[IBIS Ver]   3.2
[File Name]   sprm191a.ibs
[File Rev]   0.1
[Date]   April 20, 2006
[Source]   File Originated at Texas Instruments
[Disclaimer]   Please be aware that in the absence of a written agreement
|   Texas Instruments(TI) assumes no liability for:
|   (1) The accuracy of the IBIS models provided to your company
|   (2) The proper functioning of these Models in your design
|   or for any resulting applications;or
|   (3) Infringement of patents,copyrights, or intellectual
|   property rights resulting from your use of these models.
|   TI provides IBIS Models as a service to our customers and
|   therefore reserves the right to limit distribution of the
|   Models.
[Copyright]   Property of Texas Instruments Incorporated.
|   Unauthorized reproduction and/or distribution is strictly
|   prohibited.
|   This product is protected under copyright law and trade
|   secret law as an unpublished work.
|   Created 1999,(C) Copyright 1999-2000,
|   Texas Instruments Incorporated., All Rights Reserved.
|   These commodities are under the U.S.
|   Government distribution license control.As such,they are not
|   to be re-exported without the prior approval of the U.S.
|   Department of Commerce.
[Component]   c6727_gdh
[Manufacturer]   Texas Instruments
[Package]
|Variable   Typ   Min   Max
R_pkg   3.500e-01   2.78346e-01  4.67972e-01
L_pkg   4.000e-09   2.63574e-09  6.33212e-09
C_pkg   4.300e-013  3.00224E-013 6.87584E-013
[Pin]   signal_name   model_name
C2   AHCLKX0   BC3325BSHY
C1   AMUTE0   BC3325BSHY
C3   HD[23]   BC3325BSHYPD
D2   AMUTE1   BC3325BSHY
D1   AHCLKX1   BC3325BSHY
D3   HD[22]   BC3325BSHYPD
E2   ACLKX1   BC3325BSHY
E1   ACLKR1   BC3325BSHY
E3   HD[21]   BC3325BSHYPD
F2   AFSX1   BC3325BSHY
F1   AFSR1   BC3325BSHY
F4   HD[20]   BC3325BSHYPD
F3   HD[19]   BC3325BSHYPD
G2   RESET   IC33SHY
G4   HD[18]   BC3325BSHYPD
G3   HD[17]   BC3325BSHYPD
H2   CLKIN   IC33SHY
H1   HD[16]   BC3325BSHYPD
H4   HD[31]   BC3325BSHYPD
K3   TMS   IC33SHYPU
K4   TRST   IC33SPD
L2   HD[30]   BC3325BSHYPD
L1   TDI   IC33SHYPU
M2   TDO   BC3325BSHYPU
L4   HD[29]   BC3325BSHYPD
L3   HD[28]   BC3325BSHYPD
M1   EMU0   BC3325BSHYPU
M3   HD[27]   BC3325BSHYPD
N3   HD[26]   BC3325BSHYPD
N1   EMU1   BC3325BSHYPU
N2   HD[25]   BC3325BSHYPD
P1   TCK   IC33SHYPU
P2   HD[24]   BC3325BSHYPD
R2   EM_D[23]   BC3325BSHYPD
N4   EM_D[22]   BC3325BSHYPD
R3   SDRAM_CAS   BC3325BSHY
P3   EM_D[21]   BC3325BSHYPD
T3   EM_WE   BC3325BSHY
R4   EM_WE_DQM[0]   BC3325BSHY
P4   EM_D[20]   BC3325BSHYPD
T4   EM_D[7]   BC3325BSHY
R5   EM_D[6]   BC3325BSHY
P5   EM_D[19]   BC3325BSHYPD
T5   EM_D[5]   BC3325BSHY
R6   EM_D[4]   BC3325BSHY
N6   EM_D[18]   BC3325BSHYPD
P6   EM_D[17]   BC3325BSHYPD
T6   EM_D[3]   BC3325BSHY
R7   EM_D[2]   BC3325BSHY
N7   EM_D[16]   BC3325BSHYPD
P7   EM_D[31]   BC3325BSHYPD
R8   EM_D[1]   BC3325BSHY
T8   EM_D[0]   BC3325BSHY
N8   EM_D[30]   BC3325BSHYPD
N9   EM_D[29]   BC3325BSHYPD
R9   EM_D[15]   BC3325BSHY
T9   EM_D[14]   BC3325BSHY
P9   EM_D[28]   BC3325BSHYPD
N10   EM_D[27]   BC3325BSHYPD
R10   EM_D[13]   BC3325BSHY
R11   EM_D[12]   BC3325BSHY
T11   EM_D[11]   BC3325BSHY
R12   EM_D[10]   BC3325BSHY
T12   EM_D[9]   BC3325BSHY
R13   EM_D[8]   BC3325BSHY
T13   EM_WE_DQM[1]   BC3325BSHY
R14   EM_CLK   BC3325BSHY
T14   EM_SDCKE   BC3325BSHY
P12   EM_A[12]   BC3325BSHYPD
P10   EM_D[26]   BC3325BSHYPD
N11   EM_D[25]   BC3325BSHYPD
P11   EM_D[24]   BC3325BSHYPD
P13   EM_WE_DQM[2]   BC3325BSHYPU
R15   EM_WE_DQM[3]   BC3325BSHYPU
P14   HD[7]   BC3325BSHYPD
P15   EM_A[11]   BC3325BSHY
N14   HD[6]   BC3325BSHYPD
P16   EM_A[9]   BC3325BSHY
N15   EM_A[8]   BC3325BSHY
N13   HD[5]   BC3325BSHYPD
N16   EM_A[7]   BC3325BSHY
M15   EM_A[6]   BC3325BSHY
L14   HD[4]   BC3325BSHYPD
M16   EM_A[5]   BC3325BSHY
L15   EM_A[4]   BC3325BSHY
L13   HD[3]   BC3325BSHYPD
M14   HD[2]   BC3325BSHYPD
L16   EM_A[3]   BC3325BSHY
K15   EM_A[2]   BC3325BSHY
K14   HD[1]   BC3325BSHYPD
K13   HD[0]   BC3325BSHYPD
J15   EM_A[1]   BC3325BSHY
J16   EM_A[0]   BC3325BSHY
J13   HD[15]   BC3325BSHYPD
H13   HD[14]   BC3325BSHYPD
H15   EM_A[10]   BC3325BSHY
H16   EM_BA[1]   BC3325BSHY
H14   HD[13]   BC3325BSHYPD
G13   HD[12]   BC3325BSHYPD
G15   EM_BA[0]   BC3325BSHY
F15   EM_CS[0]   BC3325BSHY
G14   HD[11]   BC3325BSHYPD
F16   SDRAM_RAS   BC3325BSHY
E15   EM_CS[1]   BC3325BSHY
F13   HD[10]   BC3325BSHYPD
E16   EM_RNW   BC3325BSHY
D15   EM_OE   BC3325BSHY
F14   HD[9]   BC3325BSHYPD
D16   SPI0_ENA   BC3325BSHY
E14   HD[8]   BC3325BSHYPD
C15   SPI0_SCS   BC3325BSHY
D14   EM_WAIT   BC3325BSHYPU
C16   SPI0_SCLK   BC3325BSHY
C14   AHCLKR2   BC3325BSHYPD
C13   ACLKR2   BC3325BSHYPD
C12   AFSR2   BC3325BSHYPD
B15   SPI0_SIMO   BC3325BSHY
B14   SPI0_SOMI   BC3325BSHY
A14   AXR0[0]   BC3325BSHY
B13   AXR0[1]   BC3325BSHY
A13   AXR0[2]   BC3325BSHY
B12   AXR0[3]   BC3325BSHY
D11   ACLKX2   BC3325BSHYPD
A12   AXR0[4]   BC3325BSHY
B11   AXR0[5]   BC3325BSHY
C11   AFSX2   BC3325BSHYPD
D10   AMUTE2   BC3325BSHYPD
A11   AXR0[6]   BC3325BSHY
B10   AXR0[7]   BC3325BSHY
C10   HCNTL1   BC3325BSHYPD
D9   HCNTL0   BC3325BSHYPD
B9   AXR0[8]   BC3325BSHY
A9   AXR0[9]   BC3325BSHY
C9   HAS   BC3325BSHYPD
D8   HRWN   BC3325BSHYPD
B8   AXR0[10]   BC3325BSHY
A8   AXR0[11]   BC3325BSHY
C8   HCS   BC3325BSHYPU
D7   HDS1   BC3325BSHYPU
B7   AXR0[12]   BC3325BSHY
B6   AXR0[13]   BC3325BSHY
C7   HDS2   BC3325BSHYPU
A6   AXR0[14]   BC3325BSHY
B5   AXR0[15]   BC3325BSHY
D6   HRDY   BC3325BSHYPD
A5   ACLKR0   BC3325BSHY
B4   AFSR0   BC3325BSHY
C6   HBE[0]   BC3325BSHYPD
A4   ACLKX0   BC3325BSHY
C5   HBE[1]   BC3325BSHYPD
B3   AHCLKR0   BC3325BSHY
C4   HBE[2]   BC3325BSHYPD
A3   AFSX0   BC3325BSHY
B2   HBE[3]   BC3325BSHYPD
[Package Model]   BGA
[Define Package Model]  BGA
[Manufacturer]   Texas Instruments
[OEM]   Texas Instruments
[Description]   BGA
[Number Of Sections]  1
[Number Of Pins]  152
[Pin Numbers]
C2   Len=0  R=0.339392   L=3.99674e-09  C=4.70683E-013 /
C1   Len=0  R=0.387574   L=4.72766e-09  C=4.57896E-013 /
C3   Len=0  R=0.354062   L=4.32098e-09  C=4.78888E-013 /
D2   Len=0  R=0.355048   L=4.40226e-09  C=4.28982E-013 /
D1   Len=0  R=0.373336   L=5.0292e-09   C=4.24207E-013 /
D3   Len=0  R=0.33615   L=4.05326e-09  C=4.47644E-013 /
E2   Len=0  R=0.340312   L=3.9161e-09   C=4.31444E-013 /
E1   Len=0  R=0.37303   L=4.38348e-09  C=4.04001E-013 /
E3   Len=0  R=0.317216   L=3.59786e-09  C=4.63371E-013 /
F2   Len=0  R=0.349102   L=3.8723e-09   C=3.79014E-013 /
F1   Len=0  R=0.387412   L=4.62594e-09  C=3.44324E-013 /
F4   Len=0  R=0.302866   L=3.27248e-09  C=4.13775E-013 /
F3   Len=0  R=0.309298   L=3.60524e-09  C=4.51108E-013 /
G2   Len=0  R=0.40644   L=4.74502e-09  C=4.38027E-013 /
G4   Len=0  R=0.323936   L=3.67236e-09  C=5.59319E-013 /
G3   Len=0  R=0.363316   L=4.41228e-09  C=4.25543E-013 /
H2   Len=0  R=0.331636   L=4.17322e-09  C=3.77069E-013 /
H1   Len=0  R=0.3734   L=4.74898e-09  C=3.37117E-013 /
H4   Len=0  R=0.305394   L=3.38732e-09  C=4.11321E-013 /
K3   Len=0  R=0.34395   L=4.19168e-09  C=4.19243E-013 /
K4   Len=0  R=0.323068   L=3.56512e-09  C=4.53466E-013 /
L2   Len=0  R=0.415648   L=4.82438e-09  C=4.10039E-013 /
L1   Len=0  R=0.36658   L=4.26388e-09  C=3.37108E-013 /
M2   Len=0  R=0.351496   L=3.77214e-09  C=4.40172E-013 /
L4   Len=0  R=0.29318   L=3.0961e-09   C=4.23678E-013 /
L3   Len=0  R=0.303374   L=3.5041e-09   C=3.70824E-013 /
M1   Len=0  R=0.381336   L=4.89728e-09  C=3.42681E-013 /
M3   Len=0  R=0.30869   L=3.78928e-09  C=4.25211E-013 /
N3   Len=0  R=0.354404   L=4.79456e-09  C=4.88341E-013 /
N1   Len=0  R=0.377298   L=5.26052e-09  C=3.88177E-013 /
N2   Len=0  R=0.354446   L=4.67068e-09  C=4.40298E-013 /
P1   Len=0  R=0.39216   L=5.42366e-09  C=4.70847E-013 /
P2   Len=0  R=0.33903   L=4.33112e-09  C=4.85018E-013 /
R2   Len=0  R=0.358758   L=4.69614e-09  C=5.20436E-013 /
P3   Len=0  R=0.317008   L=3.1663e-09   C=5.79127E-013 /
R3   Len=0  R=0.377564   L=4.6553e-09   C=5.21684E-013 /
P4   Len=0  R=0.334572   L=4.1666e-09   C=5.00816E-013 /
T3   Len=0  R=0.39423   L=4.83226e-09  C=4.65868E-013 /
R4   Len=0  R=0.348864   L=4.1244e-09   C=4.5167E-013 /
P5   Len=0  R=0.318642   L=3.77818e-09  C=4.86875E-013 /
T4   Len=0  R=0.383618   L=4.47018e-09  C=4.83017E-013 /
R5   Len=0  R=0.340902   L=3.80248e-09  C=4.68627E-013 /
N6   Len=0  R=0.338592   L=4.07018e-09  C=5.02179E-013 /
T5   Len=0  R=0.377266   L=4.8863e-09   C=4.05001E-013 /
R6   Len=0  R=0.396836   L=4.96212e-09  C=4.46027E-013 /
P6   Len=0  R=0.284454   L=3.0839e-09   C=4.56304E-013 /
N7   Len=0  R=0.343606   L=4.04324e-09  C=5.01509E-013 /
T6   Len=0  R=0.367898   L=4.60384e-09  C=3.44563E-013 /
R7   Len=0  R=0.382064   L=4.85522e-09  C=4.38861E-013 /
P7   Len=0  R=0.304548   L=3.55168e-09  C=5.16335E-013 /
N8   Len=0  R=0.345366   L=4.34114e-09  C=4.66695E-013 /
R8   Len=0  R=0.374476   L=4.38938e-09  C=4.34623E-013 /
T8   Len=0  R=0.349502   L=4.05058e-09  C=3.23466E-013 /
N9   Len=0  R=0.286356   L=2.93566e-09  C=4.56363E-013 /
R9   Len=0  R=0.31836   L=3.642e-09   C=4.12715E-013 /
T9   Len=0  R=0.35189   L=4.19304e-09  C=3.70599E-013 /
P9   Len=0  R=0.286986   L=3.13788e-09  C=4.011E-013 /
N10  Len=0  R=0.298736   L=3.01978e-09  C=4.59479E-013 /
R10  Len=0  R=0.308532   L=3.57838e-09  C=4.08798E-013 /
R11  Len=0  R=0.307654   L=3.53184e-09  C=4.41997E-013 /
T11  Len=0  R=0.347386   L=4.44308e-09  C=4.11649E-013 /
R12  Len=0  R=0.326916   L=3.9885e-09   C=4.6626E-013 /
T12  Len=0  R=0.355142   L=4.45764e-09  C=4.33576E-013 /
R13  Len=0  R=0.336044   L=4.09862e-09  C=4.60055E-013 /
T13  Len=0  R=0.37393   L=4.23852e-09  C=4.58815E-013 /
R14  Len=0  R=0.351614   L=4.08646e-09  C=5.28565E-013 /
T14  Len=0  R=0.37809   L=4.5564e-09   C=4.93324E-013 /
P12  Len=0  R=0.297444   L=3.53228e-09  C=4.63846E-013 /
P10  Len=0  R=0.39935   L=5.59426e-09  C=6.87584E-013 /
N11  Len=0  R=0.355874   L=4.34494e-09  C=6.3559E-013 /
P11  Len=0  R=0.39247   L=5.28174e-09  C=6.34721E-013 /
P13  Len=0  R=0.398214   L=5.2647e-09   C=5.91166E-013 /
R15  Len=0  R=0.41964   L=4.4944e-09   C=5.41393E-013 /
P14  Len=0  R=0.353802   L=4.03244e-09  C=4.63753E-013 /
P15  Len=0  R=0.390764   L=4.98794e-09  C=5.13753E-013 /
N14  Len=0  R=0.383586   L=4.80594e-09  C=5.39901E-013 /
P16  Len=0  R=0.414816   L=5.00038e-09  C=4.07424E-013 /
N15  Len=0  R=0.435388   L=5.30096e-09  C=4.54764E-013 /
M14  Len=0  R=0.400542   L=5.23214e-09  C=5.86961E-013 /
N16  Len=0  R=0.405086   L=5.0574e-09   C=3.23989E-013 /
M15  Len=0  R=0.42635   L=5.33792e-09  C=4.20074E-013 /
L13  Len=0  R=0.309456   L=3.72312e-09  C=4.32031E-013 /
M16  Len=0  R=0.400858   L=5.16958e-09  C=3.79026E-013 /
L15  Len=0  R=0.356984   L=4.67638e-09  C=4.12267E-013 /
L14  Len=0  R=0.390396   L=5.13432e-09  C=5.45077E-013 /
K13  Len=0  R=0.440966   L=6.33212e-09  C=5.175E-013 /
L16  Len=0  R=0.3967   L=5.2994e-09   C=3.29066E-013 /
K15  Len=0  R=0.400428   L=4.8064e-09   C=4.2299E-013 /
K14  Len=0  R=0.43253   L=5.39866e-09  C=5.07689E-013 /
J13  Len=0  R=0.397262   L=4.91252e-09  C=4.7853E-013 /
J15  Len=0  R=0.334622   L=3.60426e-09  C=3.60659E-013 /
J16  Len=0  R=0.366318   L=4.17084e-09  C=3.68789E-013 /
H13  Len=0  R=0.296514   L=2.63574e-09  C=3.47293E-013 /
H15  Len=0  R=0.347474   L=3.63696e-09  C=3.6496E-013 /
H16  Len=0  R=0.387966   L=4.62782e-09  C=3.56703E-013 /
H14  Len=0  R=0.314584   L=3.5549e-09   C=4.15173E-013 /
G13  Len=0  R=0.292528   L=3.00696e-09  C=3.79816E-013 /
G15  Len=0  R=0.336178   L=3.8189e-09   C=4.0186E-013 /
F15  Len=0  R=0.373872   L=4.34952e-09  C=4.80159E-013 /
G14  Len=0  R=0.322406   L=3.52692e-09  C=4.7568E-013 /
F16  Len=0  R=0.398476   L=4.75114e-09  C=4.24914E-013 /
E15  Len=0  R=0.370362   L=4.30076e-09  C=4.56163E-013 /
F13  Len=0  R=0.307978   L=3.2259e-09   C=4.49248E-013 /
E16  Len=0  R=0.431744   L=4.6978e-09   C=4.0359E-013 /
D15  Len=0  R=0.441372   L=4.83302e-09  C=4.80547E-013 /
F14  Len=0  R=0.322668   L=3.63798e-09  C=4.62158E-013 /
D16  Len=0  R=0.400788   L=4.68854e-09  C=4.4558E-013 /
E14  Len=0  R=0.322534   L=3.70792e-09  C=4.33147E-013 /
C15  Len=0  R=0.371338   L=4.73808e-09  C=4.46122E-013 /
D14  Len=0  R=0.340548   L=3.98704e-09  C=4.30597E-013 /
C16  Len=0  R=0.418262   L=5.5125e-09   C=4.62327E-013 /
C14  Len=0  R=0.358998   L=4.33078e-09  C=4.82489E-013 /
C13  Len=0  R=0.32407   L=3.70724e-09  C=5.51319E-013 /
C12  Len=0  R=0.304854   L=3.50414e-09  C=5.56124E-013 /
B15  Len=0  R=0.389266   L=4.74152e-09  C=4.93804E-013 /
B14  Len=0  R=0.348332   L=3.97886e-09  C=4.97338E-013 /
A14  Len=0  R=0.393042   L=4.73298e-09  C=4.46663E-013 /
B13  Len=0  R=0.32416   L=3.88618e-09  C=4.27015E-013 /
A13  Len=0  R=0.385144   L=4.80134e-09  C=3.60484E-013 /
B12  Len=0  R=0.343196   L=4.16212e-09  C=3.97769E-013 /
D11  Len=0  R=0.279124   L=2.83434e-09  C=4.41764E-013 /
A12  Len=0  R=0.374556   L=4.68738e-09  C=3.96864E-013 /
B11  Len=0  R=0.327964   L=4.04244e-09  C=4.02491E-013 /
C11  Len=0  R=0.295882   L=3.52206e-09  C=4.1736E-013 /
D10  Len=0  R=0.278346   L=2.86822e-09  C=4.36434E-013 /
A11  Len=0  R=0.366008   L=4.4083e-09   C=3.96223E-013 /
B10  Len=0  R=0.396334   L=4.72896e-09  C=4.79263E-013 /
C10  Len=0  R=0.351776   L=3.99718e-09  C=4.83727E-013 /
D9   Len=0  R=0.317464   L=3.47724e-09  C=4.50408E-013 /
B9   Len=0  R=0.396522   L=4.88322e-09  C=4.17464E-013 /
A9   Len=0  R=0.351854   L=4.22988e-09  C=3.00224E-013 /
C9   Len=0  R=0.34467   L=3.99966e-09  C=4.19395E-013 /
D8   Len=0  R=0.316576   L=3.52488e-09  C=4.3496E-013 /
B8   Len=0  R=0.377636   L=4.48194e-09  C=3.68869E-013 /
A8   Len=0  R=0.349388   L=4.04516e-09  C=3.15722E-013 /
C8   Len=0  R=0.296362   L=3.39222e-09  C=4.08972E-013 /
D7   Len=0  R=0.284648   L=2.84656e-09  C=4.14454E-013 /
B7   Len=0  R=0.325322   L=3.89884e-09  C=3.78093E-013 /
B6   Len=0  R=0.397078   L=5.02496e-09  C=4.34577E-013 /
C7   Len=0  R=0.339446   L=4.10062e-09  C=4.61546E-013 /
A6   Len=0  R=0.362946   L=4.83208e-09  C=3.20462E-013 /
B5   Len=0  R=0.334594   L=4.15556e-09  C=4.13404E-013 /
D6   Len=0  R=0.28005   L=2.92398e-09  C=4.95448E-013 /
A5   Len=0  R=0.373112   L=4.48016e-09  C=3.70368E-013 /
B4   Len=0  R=0.357184   L=4.21292e-09  C=4.43331E-013 /
C6   Len=0  R=0.293942   L=3.64362e-09  C=4.31232E-013 /
A4   Len=0  R=0.394576   L=4.53714e-09  C=3.64188E-013 /
C5   Len=0  R=0.309068   L=3.49144e-09  C=3.90872E-013 /
B3   Len=0  R=0.356056   L=4.2207e-09   C=3.82479E-013 /
C4   Len=0  R=0.32827   L=3.85614e-09  C=4.45165E-013 /
A3   Len=0  R=0.389164   L=4.84752e-09  C=4.30099E-013 /
B2   Len=0  R=0.354458   L=4.1674e-09   C=6.05361E-013 /
[End_Package_Model]
[Component]   BC3325BSHY
[Manufacturer]   Texas Instruments
[Package]
|   typ   min   max
R_pkg   0   0   0
L_pkg   0   0   0
C_pkg   0   0   0
[Pin]   signal_name   model_name   R_pin   L_pin   C_pin
   1   Y   BC3325BSHY   0   0   0
[Component]   BC3325BSHYPU
[Manufacturer]   Texas Instruments
[Package]
|   typ   min   max
R_pkg   0   0   0
L_pkg   0   0   0
C_pkg   0   0   0
[Pin]   signal_name   model_name   R_pin   L_pin   C_pin
   1   Y   BC3325BSHYPU   0   0   0
[Component]   BC3325BSHYPD
[Manufacturer]   Texas Instruments
[Package]
|   typ   min   max
R_pkg   0   0   0
L_pkg   0   0   0
C_pkg   0   0   0
[Pin]   signal_name   model_name   R_pin   L_pin   C_pin
   1   Y   BC3325BSHYPD   0   0   0
[Component]   IC33SHY
[Manufacturer]   Texas Instruments
[Package]
|   typ   min   max
R_pkg   0   0   0
L_pkg   0   0   0
C_pkg   0   0   0
[Pin]   signal_name   model_name   R_pin   L_pin   C_pin
   1   A   IC33SHY   0   0   0
[Component]   IC33SHYPU
[Manufacturer]   Texas Instruments
[Package]
|   typ   min   max
R_pkg   0   0   0
L_pkg   0   0   0
C_pkg   0   0   0
[Pin]   signal_name   model_name   R_pin   L_pin   C_pin
   1   A   IC33SHYPU   0   0   0
[Component]   IC33SPD
[Manufacturer]   Texas Instruments
[Package]
|   typ   min   max
R_pkg   0   0   0
L_pkg   0   0   0
C_pkg   0   0   0
[Pin]   signal_name   model_name   R_pin   L_pin   C_pin
   1   A   IC33SPD   0   0   0
| Models and submodels in the file (6): BC3325BSHY (I/O), BC3325BSHYPU (I/O), BC3325BSHYPD (I/O), IC33SHY (Input), IC33SHYPU (Input), IC33SPD (Input)
